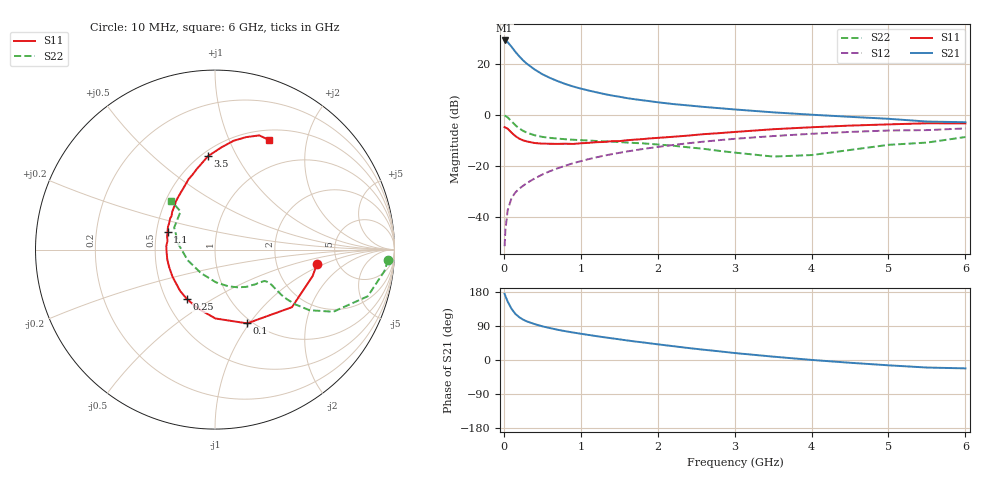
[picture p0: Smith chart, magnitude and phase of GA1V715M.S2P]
! Infineon Technologies  Discrete & RF Semiconductors
! BF775
! Si NPN RF Bipolar Junction Transistor in SOT23
! VCE = 1.75 V  IC = 15 mA
! Common Emitter S-Parameters:  May  1996
# GHz  S  MA  R  50
!  f  S11  S21  S12  S22
! GHz  MAG  ANG  MAG  ANG  MAG  ANG  MAG  ANG
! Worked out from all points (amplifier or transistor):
!   36 points, 10 MHz to 6 GHz, reference 50 ohm
!   highest |S21| = 29.1 dB at 10 MHz (marker M1)
!   |S21| within 3 dB of that: start of sweep to 113.3 MHz
!   unconditionally stable (mu >= 1): 404.3 MHz to 3.953 GHz; 5.352 GHz to 5.855 GHz
!   at 250 MHz: K = 0.84, MSG = 24.5 dB, |S12| = -27.8 dB
!   at 1.4 GHz: K = 1.13, MAG = 9.3 dB, |S12| = -15.4 dB
!   at 6 GHz: K = 1.00, MSG = 1.2 dB, |S12| = -5.3 dB
!   S11 on the Smith chart (normalised r, x): 10 MHz: 3.49, -0.81; 100 MHz: 0.95, -0.97; 250 MHz: 0.64, -0.39; 1.1 GHz: 0.57, +0.12; 3.5 GHz: 0.54, +0.77; 6 GHz: 0.62, +1.42
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0.01  0.5743 -7.8  28.44 174.5  0.0027 88.6  0.9656 -3.4
0.02  0.5638 -15.1  28.15 168.9  0.0055 82.6  0.9518 -7.2
0.05  0.5356 -36.8  26.31 154.1  0.0137 74.9  0.8897 -17.0
0.1  0.4482 -66.5  21.39 135.1  0.0235 67.5  0.7449 -27.7
0.15  0.3838 -89.6  17.05 121.6  0.0304 62.9  0.6251 -32.7
0.2  0.342 -105.9  13.94 113.0  0.0359 62.7  0.5423 -34.3
0.25  0.3171 -119.4  11.62 106.6  0.0409 62.8  0.4864 -34.6
0.3  0.3013 -130.2  9.95 101.8  0.0464 63.9  0.4474 -34.3
0.4  0.2809 -147.5  7.709 94.8  0.0569 65.3  0.3982 -32.9
0.5  0.2733 -159.6  6.225 88.9  0.0679 66.5  0.3703 -31.9
0.6  0.2715 -168.3  5.259 84.2  0.0791 66.8  0.3542 -31.6
0.8  0.2722 176.2  4.001 76.0  0.1012 66.5  0.3333 -32.0
0.9  0.2693 170.0  3.583 72.5  0.113 66.1  0.3253 -32.6
1.1  0.2824 159.4  2.992 66.2  0.1357 64.8  0.3139 -35.2
1.3  0.2942 150.5  2.558 60.1  0.1587 63.0  0.3031 -37.9
1.6  0.3186 138.4  2.12 51.7  0.1917 59.8  0.2871 -43.4
2.2  0.3719 120.6  1.624 36.5  0.2571 52.7  0.2488 -57.8
3  0.4617 102.5  1.273 18.4  0.3393 41.9  0.1825 -88.3
3.5  0.5225 94.2  1.118 8.9  0.3841 34.9  0.1526 -120.6
4.5  0.6152 80.3  0.913 -7.3  0.4628 21.1  0.2053 171.9
5.5  0.6825 68.8  0.738 -19.9  0.5022 6.7  0.2863 132.0
6  0.6807 63.7  0.716 -22.1  0.5419 2.7  0.3679 132.1
